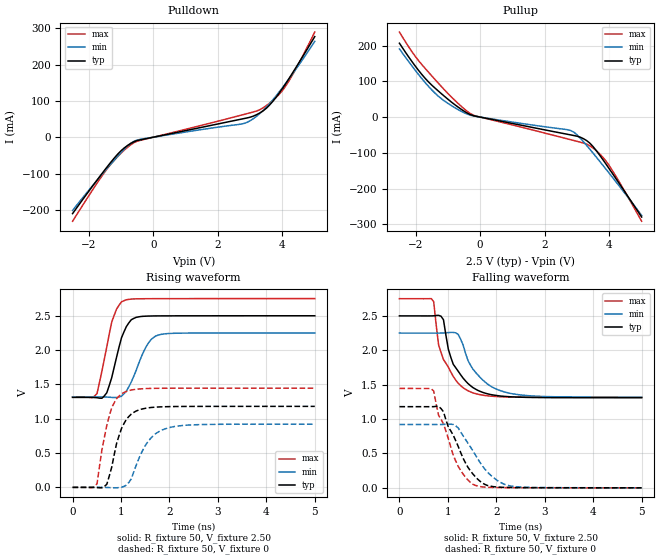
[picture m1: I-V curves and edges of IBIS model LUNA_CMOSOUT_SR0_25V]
[IBIS Ver]   3.2
[Comment Char]   |_char
[File name]   sg8201cja_25v_e.ibs
[File Rev]   1.1
[Date]   2021/10/19 9:35:58
[Source]
[Notes]
[Disclaimer]
This information is for modeling purposes only, and is not guaranteed.
Property of SEIKO EPSON Corp.,
unauthorized reproduction and/or distribution is strictly prohibited.
[Copyright]
Copyright 2021, SEIKO EPSON Corp.
[Component]   2G005_2016
Si_location Pin
Timing_location Pin
[Manufacturer]   SEIKO EPSON Corp.
| 2016 PKG
[Package]
R_pkg   25m   NA   NA
L_pkg   0.25n   NA   NA
C_pkg   0.183p   NA   NA
[Pin] signal_name   model_name
1   OE   NC
2   GND   GND
3   OUT   LUNA_CMOSOUT_SR0_25V
4   VCC   POWER
| Models and submodels in the file (1): LUNA_CMOSOUT_SR0_25V (Output)
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[Model]   LUNA_CMOSOUT_SR0_25V
Model_type Output
Polarity Non-Inverting
Vmeas=1.25
C_comp   2.5p   2.0p   3.0p
[Temperature Range] 25   140   -40
[Voltage Range]   2.50   2.25   2.75
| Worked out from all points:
|   slope of the pulldown table from 0 to 0.375 V, typ, clamps not added: 55.5 ohm
|   slope of the pullup table from 0 to 0.375 V, typ, clamps not added: 56.1 ohm
|   falling waveform, R_fixture 50, V_fixture 2.50: 20-80 % time 423ps typ, 509ps min, 383ps max; typ from 2.5 V to 1.31 V
|   falling waveform, R_fixture 50, V_fixture 0: 20-80 % time 497ps typ, 550ps min, 455ps max; typ from 1.18 V to 0.001 V
|   rising waveform, R_fixture 50, V_fixture 2.50: 20-80 % time 273ps typ, 342ps min, 259ps max; typ from 1.31 V to 2.5 V
|   rising waveform, R_fixture 50, V_fixture 0: 20-80 % time 288ps typ, 401ps min, 253ps max; typ from 0 V to 1.18 V
[Pullup]
-2.5V     206.8mA    190.9mA    238.1mA
-2V       141.6mA    129.7mA    168.8mA
-1.4V     81.31mA    67.1mA     105.4mA
-900mV    42.74mA    32.65mA    57.05mA
-300mV    6.725mA    5.122mA    9.643mA
2.8V      -49.82mA   -37.52mA   -63.25mA
3V        -53.5mA    -49.76mA   -67.91mA
3.3V      -65.99mA   -79.55mA   -75.71mA
3.6V      -94.36mA   -112.5mA   -94.49mA
3.9V      -132mA     -146.3mA   -123.4mA
4.3V      -185mA     -192.2mA   -180.4mA
5V        -279.7mA   -275.2mA   -291.6mA
[Pulldown]
-2.5V     -210.5mA   -201.8mA   -231.5mA
-1.8V     -125.1mA   -124.9mA   -134.4mA
-1.4V     -78.41mA   -82.72mA   -83.66mA
-1V       -37.44mA   -42.51mA   -44.15mA
-600mV    -12.54mA   -11.21mA   -15.17mA
2.8V      51.12mA    37.65mA    62.53mA
3.1V      58.13mA    51.19mA    69.56mA
3.4V      72.49mA    73.38mA    80.87mA
3.7V      98.59mA    102.6mA    101.3mA
4.1V      147.6mA    148.2mA    141mA
4.5V      203.8mA    198mA      202.3mA
5V        277mA      263.9mA    289.6mA
[Falling Waveform]
R_fixture=50
V_fixture=2.50
V_fixture_min=2.25
V_fixture_max=2.75
0s        2.5V       2.25V      2.75V
707.1ps   2.501V     2.25V      2.706V
808.1ps   2.508V     2.25V      2.08V
909.1ps   2.444V     2.252V     1.866V
1.01ns    2.014V     2.257V     1.754V
1.111ns   1.796V     2.26V      1.619V
1.212ns   1.696V     2.232V     1.521V
1.465ns   1.486V     1.786V     1.396V
2.323ns   1.323V     1.369V     1.319V
5ns       1.311V     1.318V     1.316V
[Falling Waveform]
R_fixture=50
V_fixture=0
V_fixture_min=0
V_fixture_max=0
0s        1.18V      920.9mV    1.445V
707.1ps   1.181V     920.6mV    1.409V
808.1ps   1.183V     920.4mV    1.055V
909.1ps   1.106V     921.9mV    930mV
1.162ns   685.8mV    901.1mV    391.2mV
1.364ns   362.7mV    703.6mV    156.2mV
1.566ns   162.7mV    481.3mV    37.43mV
1.869ns   26.01mV    194mV      7.064mV
2.273ns   5.653mV    30.35mV    2.84mV
5ns       646.8uV    1.134mV    412.8uV
[Rising Waveform]
R_fixture=50
V_fixture=2.50
V_fixture_min=2.25
V_fixture_max=2.75
0s        1.311V     1.317V     1.316V
505.1ps   1.306V     1.318V     1.366V
707.1ps   1.378V     1.316V     2.048V
808.1ps   1.598V     1.311V     2.407V
909.1ps   1.898V     1.309V     2.597V
1.061ns   2.264V     1.362V     2.719V
1.212ns   2.442V     1.535V     2.743V
1.515ns   2.495V     2.046V     2.748V
1.768ns   2.498V     2.218V     2.749V
5ns       2.5V       2.25V      2.75V
[Rising Waveform]
R_fixture=50
V_fixture=0
V_fixture_min=0
V_fixture_max=0
0s        0V         554.8nV    0V
505.1ps   -3.02mV    271.1uV    52.65mV
606.1ps   -5.941mV   376.1uV    546.4mV
707.1ps   45.59mV    -1.33mV    904.3mV
808.1ps   293.5mV    -4.91mV    1.162V
909.1ps   640.1mV    -6.688mV   1.293V
1.111ns   991.9mV    33.02mV    1.398V
1.515ns   1.153V     624.8mV    1.44V
1.919ns   1.175V     855mV      1.444V
5ns       1.18V      920.8mV    1.445V
[Ramp]
R_load=50
dV/dt_r   7.082E-1/2.843E-10   5.525E-1/4.009E-10   8.670E-1/2.514E-10
dV/dt_f   7.137E-1/4.220E-10   5.594E-1/5.090E-10   8.606E-1/3.830E-10
|[End   LUNA_CMOSOUT_SR0_25V
